{attribute 'hide_all_locals'}
FUNCTION_BLOCK FB_Pulse
VAR_INPUT
	IN				:	BOOL;
	PT_ON			:	TIME;
	PT_OFF			:	TIME;
END_VAR
VAR_OUTPUT
	Q				:	BOOL;
	RT				:	BOOL;
	FT				:	BOOL;
END_VAR
VAR
	R_T				:	R_TRIG;
	TON_ON			:	TON;
	TON_OFF			:	TON;
	_TempBool		:	BOOL;
	_Q				:	BOOL;
END_VAR

RT := FT := FALSE;
IF NOT IN THEN 
	R_T(CLK:= FALSE);
	TON_ON(IN:= FALSE);
	TON_OFF(IN:= FALSE);
	_TempBool := FALSE;	
	Q := FALSE;
ELSE
	R_T(CLK:= TRUE, Q=> RT);
	IF NOT _TempBool THEN 
		TON_ON(IN:= TRUE, PT:= PT_OFF, Q=> , ET=> );
		TON_OFF(IN:= FALSE, PT:= PT_ON, Q=> , ET=> );
		_TempBool := TON_ON.Q;
		FT := _TempBool;
		Q := TRUE;
	ELSE
		TON_ON(IN:= FALSE, PT:= PT_OFF, Q=> , ET=> );
		TON_OFF(IN:= TRUE, PT:= PT_ON, Q=>  , ET=> );
		_TempBool := NOT TON_OFF.Q;
		RT := NOT _TempBool;
		Q := FALSE;
	END_IF
END_IF

END_FUNCTION_BLOCK
